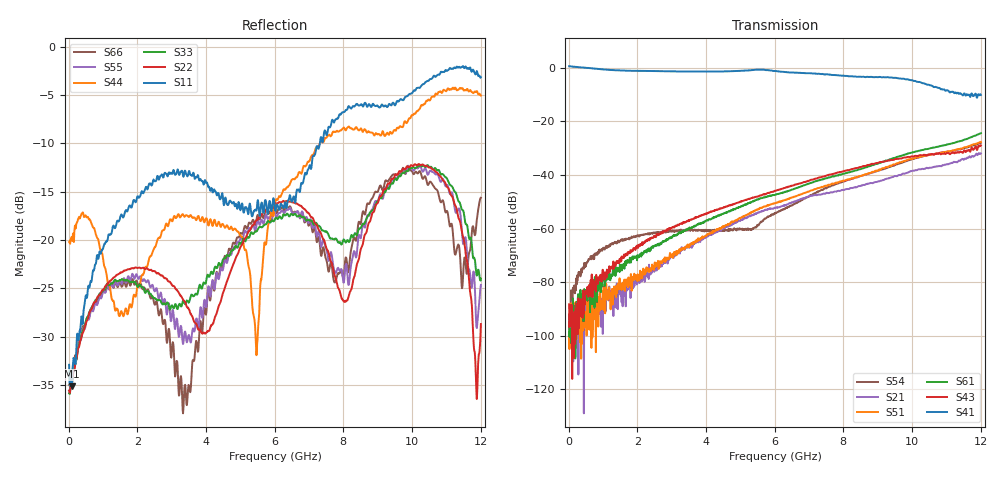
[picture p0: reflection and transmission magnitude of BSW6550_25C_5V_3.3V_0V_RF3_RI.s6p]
! Agilent Technologies	N5230C	MY49001333	A.09.33.09
!	Test time	=	2026-05-06 10:00
!	Product	=	BSW6550
!	Temp	=	25C
!	VDD	=	5
!	Control_High	=	3.3
!	Control_Low	=	0
!	Logic	=	RF3
!	Port1	=	RFC
!	Port2	=	RF1
!	Port3	=	RF2
!	Port4	=	RF3
!	Port5	=	RF4
!	Port6	=	RF5
!	V1	=	3.3 / 0
!	V2	=	3.3 / 0
!	V3	=	3.3 / 0
!S6P File: Measurements: <S11,S12,S13,S14,S15,S16>,
!<S21,S22,S23,S24,S25,S26>,
!<S31,S32,S33,S34,S35,S36>,
!<S41,S42,S43,S44,S45,S46>,
!<S51,S52,S53,S54,S55,S56>,
!<S61,S62,S63,S64,S65,S66>;
# HZ S RI R 50
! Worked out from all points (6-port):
!   1201 points, 10 MHz to 12.01 GHz, reference 50 ohm
!   strongest paths, dB at 10 MHz, 3.01 GHz, 6.01 GHz, 9.01 GHz, 12.01 GHz:
!     S41: 0.6, -1.3, -1.2, -3.5, -10.1
!     S43: -88.2, -59.6, -45.9, -35.5, -29.0
!     S61: -100.2, -63.4, -47.5, -35.8, -24.4
!     S51: -95.9, -70.1, -50.5, -38.3, -27.7
!     S21: -94.7, -70.6, -52.2, -42.4, -32.0
!     S54: -97.3, -61.1, -54.3, -38.5, -28.0
!   lowest |S11| = -35.2 dB at 90 MHz (marker M1), VSWR 1.04, Z = 51.7 - j0.593 ohm
!   |S11| at or under -10 dB: start of sweep to 7.316 GHz
